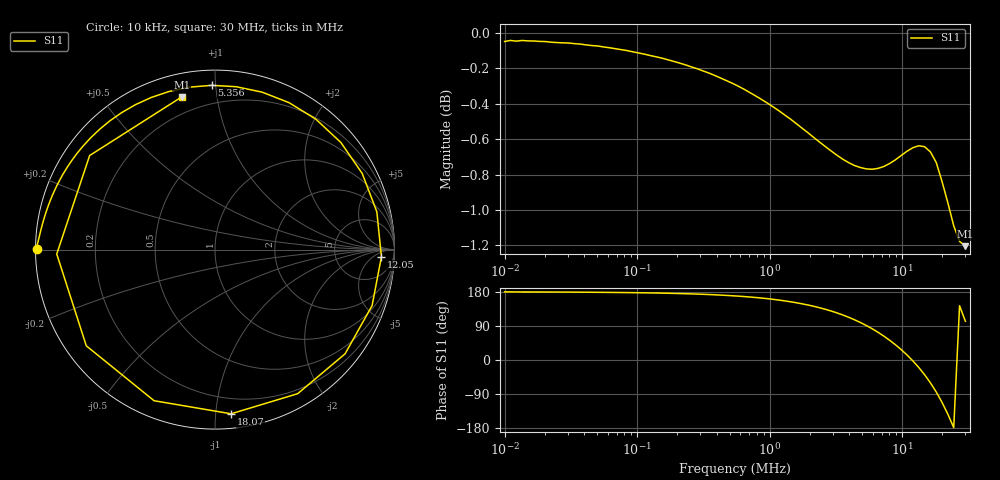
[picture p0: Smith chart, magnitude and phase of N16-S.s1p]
! ListType=Log
!!2-Port #16 Magnet Short
# MHz S RI R 50
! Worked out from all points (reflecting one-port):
!   80 points, 10 kHz to 30 MHz, reference 50 ohm
!   lowest |S11| = -1.2 dB at 30 MHz (marker M1), VSWR 14.44, Z = 5.69 + j39.9 ohm
!   phase of S11 starts at 180 deg and turns -437 deg over the sweep
!   S11 on the Smith chart (normalised r, x): 10 kHz: 0.00, +0.00; 5.356 MHz: 0.09, +0.98; 12.05 MHz: 20, -12; 18.07 MHz: 0.09, -1.10; 30 MHz: 0.11, +0.80
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0.01  -0.9945 0.00384
0.0275513  -0.9935 0.0135
0.0759074  -0.9886 0.0335
0.2091346  -0.9774 0.0794
0.5761927  -0.947 0.1911
0.9563981  -0.9083 0.2967
1.587485  -0.8255 0.4553
2.151554  -0.7332 0.5791
2.635  -0.6424 0.6708
3.571274  -0.4424 0.8079
4.373726  -0.2549 0.8812
5.356486  -0.0181 0.9152
6.560068  0.2626 0.8772
7.259765  0.4129 0.8185
8.034091  0.5622 0.7264
8.891007  0.7019 0.596
9.839321  0.8203 0.4239
10.88878  0.9018 0.2101
12.05018  0.9272 -0.0397
13.33545  0.8753 -0.312
14.75781  0.7246 -0.5809
16.33188  0.4607 -0.8027
18.07383  0.0899 -0.9148
20.00159  -0.3393 -0.842
22.13496  -0.7171 -0.5361
24.49587  -0.8817 -0.0246
27.1086  -0.6984 0.5241
30  -0.1857 0.8504
